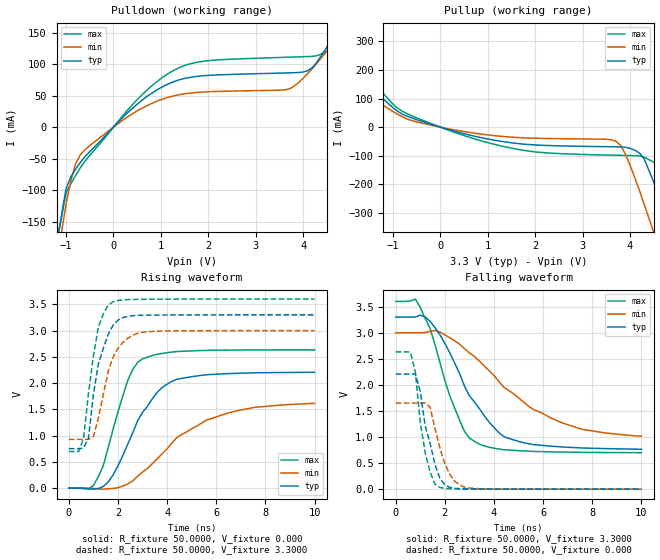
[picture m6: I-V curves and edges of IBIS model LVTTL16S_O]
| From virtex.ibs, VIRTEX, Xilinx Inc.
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|   Model LVTTL16S_O
[Model]   LVTTL16S_O
Model_type   Output
Polarity   Non-Inverting
Vmeas =   1.4000V
Cref =  35.0000pF
Rref =   1.0000M
Vref =  0.000V
C_comp   6.5000pF   5.0000pF   8.0000pF
[Temperature Range]   27.0000   100.0000   0.000
[Voltage Range]   3.3000V   3.0000V   3.6000V
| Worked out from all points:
|   slope of the pulldown table from 0 to 0.495 V, typ, clamps not added: 13.7 ohm
|   slope of the pullup table from 0 to 0.495 V, typ, clamps not added: 21.7 ohm
|   rising waveform, R_fixture 50.0000, V_fixture 0.000: 20-80 % time 1.49ns typ, 2.54ns min, 994ps max; typ from 0 V to 2.21 V
|   rising waveform, R_fixture 50.0000, V_fixture 3.3000: 20-80 % time 623ps typ, 703ps min, 506ps max; typ from 0.751 V to 3.3 V
|   falling waveform, R_fixture 50.0000, V_fixture 3.3000: 20-80 % time 1.82ns typ, 3.1ns min, 1.2ns max; typ from 3.3 V to 0.766 V
|   falling waveform, R_fixture 50.0000, V_fixture 0.000: 20-80 % time 590ps typ, 632ps min, 465ps max; typ from 2.21 V to 0 V
[Pulldown]
| voltage   I(typ)   I(min)   I(max)
-3.3V     -1.282A    -1.27A     -1.284A
-1.5V     -319.5mA   -354.4mA   -307.2mA
-1V       -97.76mA   -122.6mA   -104.7mA
-800mV    -66.75mA   -58.46mA   -76.88mA
-600mV    -46.92mA   -35.82mA   -53.89mA
600mV     42.55mA    29.94mA    51.16mA
1.4V      75.27mA    51.64mA    94.7mA
3.7V      86.04mA    60.44mA    110.9mA
4.1V      89.48mA    85.22mA    111.9mA
4.5V      126.6mA    120.5mA    120.3mA
4.9V      177.6mA    159.9mA    174.2mA
6.6V      407.8mA    336.3mA    452.6mA
[Pullup]
| voltage   I(typ)   I(min)   I(max)
-3.3V     413.8mA    317.9mA    498.5mA
-2.9V     356.6mA    273mA      429.3mA
-2.5V     297.6mA    226.1mA    358.6mA
-600mV    31.98mA    22.96mA    39.44mA
1.5V      -54.66mA   -34.94mA   -73.46mA
3.7V      -68.75mA   -48.9mA    -98.25mA
3.9V      -70.27mA   -93.43mA   -98.9mA
4.2V      -90.62mA   -222.7mA   -100.8mA
4.5V      -192.3mA   -368.3mA   -122.6mA
4.9V      -393.7mA   -569.2mA   -241mA
5.1V      -499.3mA   -670.9mA   -340.5mA
6.6V      -1.31A     -1.442A    -1.157A
[Ramp]
| variable   typ   min   max
dV/dt_r   1.3230/1.4802n   0.9678/2.6002n   1.5792/0.9791n
dV/dt_f   1.5203/1.8143n   1.1904/3.0557n   1.7401/1.1989n
R_load = 50.0000
[Rising Waveform]
R_fixture = 50.0000
V_fixture = 0.000
| time   V(typ)   V(min)   V(max)
0s        0V         0V         0V
1ns       -18.21mV   -4.471mV   51.88mV
1.4ns     30.55mV    -19.12mV   428.3mV
1.8ns     250.3mV    -5.929mV   1.121V
2.4ns     838.6mV    82.03mV    2.052V
3ns       1.443V     308.1mV    2.462V
4.2ns     2.034V     862.1mV    2.591V
5.6ns     2.158V     1.294V     2.623V
7.6ns     2.196V     1.54V      2.631V
10ns      2.205V     1.613V     2.632V
[Rising Waveform]
R_fixture = 50.0000
V_fixture = 3.3000
V_fixture_min = 3.0000
V_fixture_max = 3.6000
| time   V(typ)   V(min)   V(max)
0s        751.2mV    928.2mV    696.8mV
400ps     751.8mV    928.3mV    698.3mV
600ps     761.4mV    928.7mV    946.2mV
800ps     949.3mV    928.5mV    1.807V
1ns       1.782V     982.8mV    2.51V
1.2ns     2.361V     1.326V     3.067V
1.8ns     3.102V     2.491V     3.548V
2.4ns     3.271V     2.854V     3.588V
3ns       3.291V     2.967V     3.594V
10ns      3.299V     2.999V     3.599V
[Falling Waveform]
R_fixture = 50.0000
V_fixture = 3.3000
V_fixture_min = 3.0000
V_fixture_max = 3.6000
| time   V(typ)   V(min)   V(max)
0s        3.3V       3V         3.6V
800ps     3.302V     3V         3.645V
1ns       3.337V     2.999V     3.485V
1.8ns     2.959V     3.013V     2.428V
2.6ns     2.219V     2.781V     1.323V
3.2ns     1.675V     2.547V     918.8mV
4.2ns     1.084V     2.066V     769.7mV
5ns       916.2mV    1.748V     738.8mV
7.4ns     793.9mV    1.174V     707mV
10ns      766.2mV    1.016V     699.9mV
[Falling Waveform]
R_fixture = 50.0000
V_fixture = 0.000
| time   V(typ)   V(min)   V(max)
0s        2.208V     1.651V     2.633V
600ps     2.208V     1.651V     2.628V
800ps     2.209V     1.651V     2.242V
1ns       1.878V     1.65V      1.285V
1.2ns     1.216V     1.653V     697.4mV
1.4ns     876.5mV    1.571V     330.3mV
1.8ns     204.8mV    784mV      32.62mV
2.2ns     34.88mV    284.6mV    9.219mV
2.8ns     6.162mV    39.2mV     3.371mV
10ns      337.3uV    476.1uV    290.3uV
